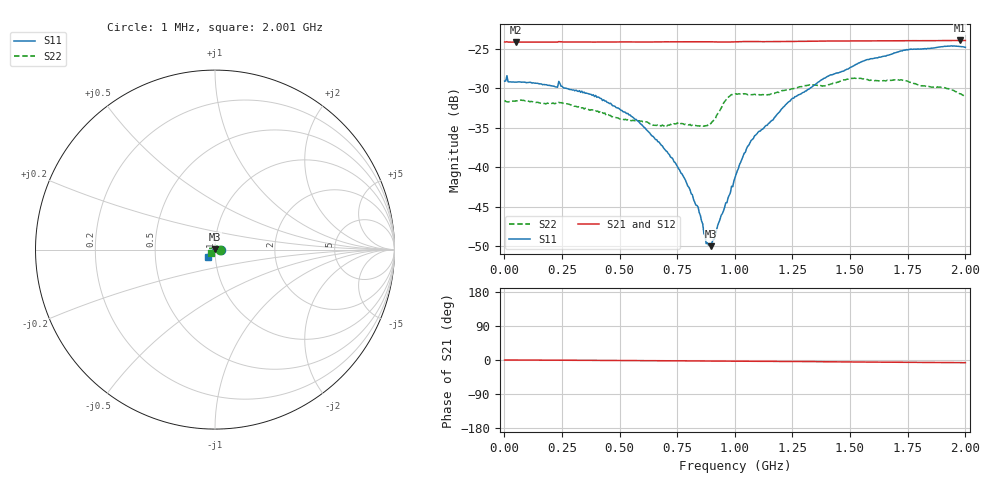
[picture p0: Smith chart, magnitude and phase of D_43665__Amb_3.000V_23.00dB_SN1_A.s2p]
! device id: 43665_
! dir: \\malibu\benchdata\1_engineers\tn_data\43665_75ohm\new\sparar\43665_\amb\3p000v\23p00db
! Serial: 1
! Insertion: A
! Temp: Amb
! VDD: 3.000V
! Attenuation Step: 23.00dB
! IDD: 1.451141e+00mA
! FILE NAME
! DATE 03-27-2009 08:39:00
! CORRECTED  DATA
#  Hz  S  RI  R  75
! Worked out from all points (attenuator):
!   401 points, 1 MHz to 2.001 GHz, reference 75 ohm
!   highest |S21| = -23.96 dB at 1.976 GHz (marker M1); lowest = -24.2 dB at 51 MHz (marker M2)
!   lowest |S11| = -50.0 dB at 896 MHz (marker M3), VSWR 1.01, Z = 74.7 + j0.381 ohm
!   |S11| at or under -10 dB: start of sweep to end of sweep
!   |S22| runs from -34.8 to -28.7 dB; largest |S21 - S12| = 0.00042
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1000000  0.0351 -0.000276  0.062 -0.000122  0.0621 -0.00013  0.0265 -0.000298
5.1e7  0.0345 0.00102  0.0618 -0.000112  0.0619 -0.000104  0.0262 0.00246
2.46e8  0.0323 0.00447  0.062 -0.000615  0.0619 -0.000601  0.0222 0.0128
3.36e8  0.0298 0.00556  0.062 -0.000913  0.062 -0.000858  0.0173 0.0163
5.46e8  0.0201 0.00727  0.062 -0.0016  0.062 -0.00154  0.00517 0.0192
6.71e8  0.0129 0.00652  0.062 -0.00194  0.0621 -0.00183  -0.00282 0.0181
7.81e8  0.00665 0.00538  0.0621 -0.00243  0.0622 -0.00229  -0.0101 0.0157
8.46e8  0.00244 0.00455  0.0622 -0.00271  0.0622 -0.00264  -0.0139 0.0118
8.76e8  -0.000328 0.00327  0.0621 -0.00292  0.0622 -0.00276  -0.0158 0.00925
8.96e8  -0.00189 0.00255  0.0621 -0.00304  0.0621 -0.00285  -0.0172 0.00792
9.06e8  -0.00269 0.0022  0.062 -0.00307  0.0621 -0.0029  -0.0182 0.00735
9.61e8  -0.00593 0.000636  0.0619 -0.00309  0.0619 -0.00289  -0.0258 0.00633
1.001e9  -0.00858 -3.78e-05  0.062 -0.00304  0.0621 -0.00285  -0.028 0.00779
1.046e9  -0.0124 -0.00135  0.0623 -0.00331  0.0623 -0.0031  -0.0285 0.00607
1.096e9  -0.0158 -0.00385  0.0623 -0.00374  0.0624 -0.00351  -0.0286 0.00387
1.241e9  -0.0244 -0.00974  0.0623 -0.00419  0.0625 -0.00394  -0.0308 -0.00427
1.336e9  -0.0288 -0.0145  0.0626 -0.00463  0.0627 -0.00433  -0.032 -0.00887
1.546e9  -0.0379 -0.0264  0.0626 -0.00576  0.0629 -0.00557  -0.0316 -0.0183
1.671e9  -0.04 -0.0323  0.0627 -0.00639  0.0629 -0.00621  -0.0293 -0.0197
1.756e9  -0.0409 -0.0376  0.0628 -0.00677  0.063 -0.00667  -0.0265 -0.0222
1.976e9  -0.0382 -0.0436  0.0629 -0.00773  0.0631 -0.00769  -0.0207 -0.0206
2.001e9  -0.0376 -0.0433  0.0629 -0.00776  0.063 -0.00778  -0.0196 -0.0198
